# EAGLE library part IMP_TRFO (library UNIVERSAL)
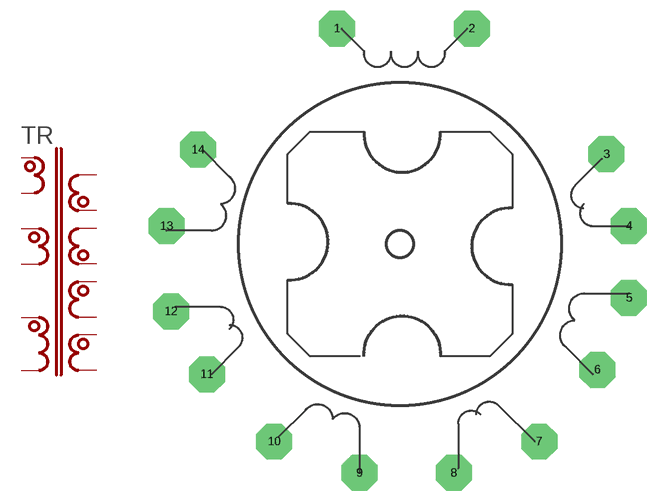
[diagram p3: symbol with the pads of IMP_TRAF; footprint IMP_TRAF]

Designator prefix TR

## IMP_TRFO  [IMP_TRAF]
1  1
2  2
3  3
4  4
5  5
6  6
7  7
8  8
9  9
10  10
11  11
12  12
13  13
14  14

## Footprint IMP_TRAF (pad centres in mm)
drill 0.813 pad 5.08 octagon: 1 -8.89,30.48; 2 10.16,30.48; 3 29.21,12.7; 4 32.385,2.54; 5 32.385,-7.62; 6 27.94,-17.78; 7 19.685,-27.94; 8 7.62,-32.385; 9 -5.715,-32.385; 10 -17.78,-27.94; 11 -27.305,-18.415; 12 -32.385,-9.525; 13 -33.02,2.54; 14 -28.575,13.335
